(* Logix 5000 AddOnInstructionDefinition export Banner_QS18E_Param_v4; software revision 33.00; part 2 of 3 *)
(* tags used below, declared in another part *)
   QS18E : Banner_QS18E_v4;
   Port_Data : Banner_IOL_Port_v4;
   Port : DINT;
   Sensor_Type : DINT;   // 1 = D, DV, LP, CV, & FP models, 2 = EV or E models, 3 = RV or R models.
   Local_Control : DINT;
   Command_Being_Processed : BOOL;
   Update_Archive : BOOL;
   Index_Write_Inprocess : INT;
   Index_Write_Control : INT;
   Inprocess_Index : DINT;
(* Banner_QS18E_Param_v4, continued *)

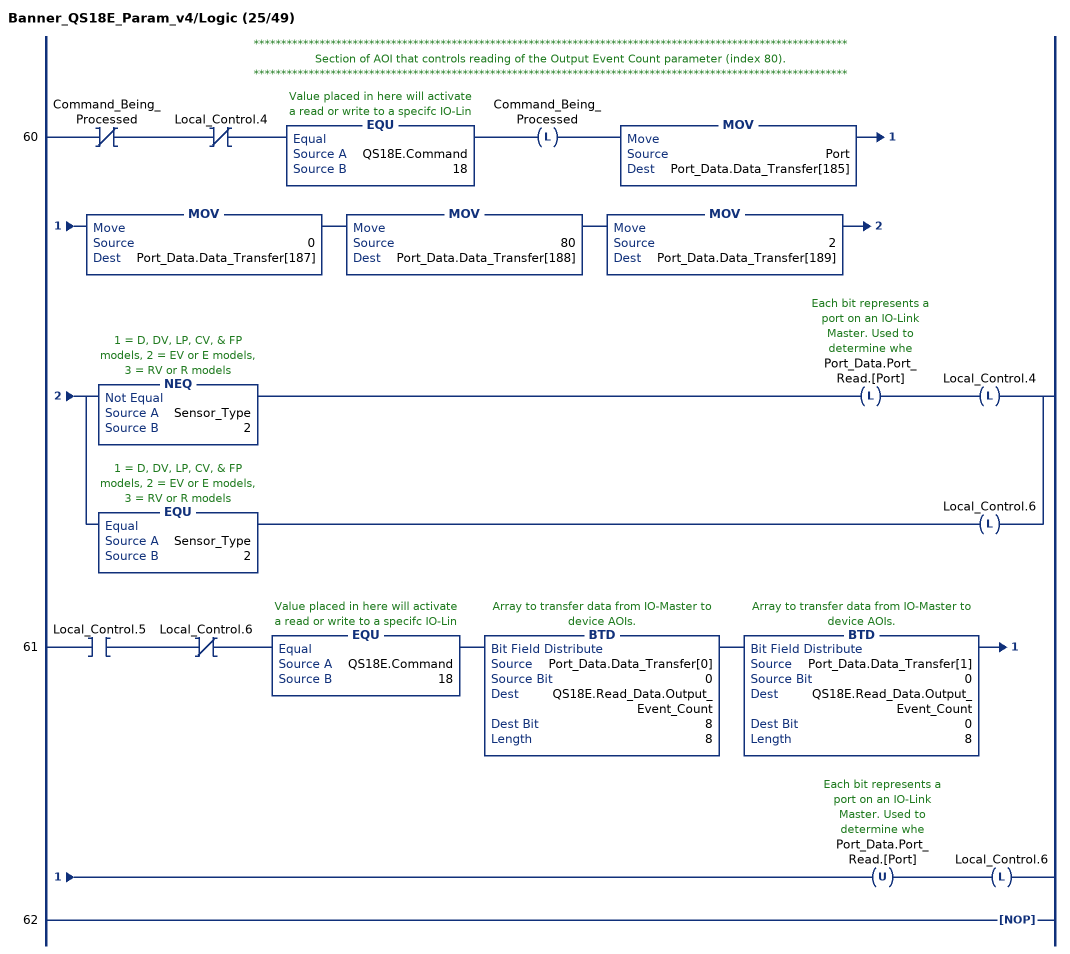
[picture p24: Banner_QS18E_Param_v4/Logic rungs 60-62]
   // ************************************************************************************************************
   // Section of AOI that controls reading of the Output Event Count parameter (index 80).
   // ************************************************************************************************************
   60: XIO(Command_Being_Processed)XIO(Local_Control.4)EQU(QS18E.Command,18)OTL(Command_Being_Processed)MOV(Port,Port_Data.Data_Transfer[185])MOV(0,Port_Data.Data_Transfer[187])MOV(80,Port_Data.Data_Transfer[188])MOV(2,Port_Data.Data_Transfer[189])[NEQ(Sensor_Type,2) OTL(Port_Data.Port_Read.[Port]) OTL(Local_Control.4) ,EQU(Sensor_Type,2) OTL(Local_Control.6) ];
   61: XIC(Local_Control.5)XIO(Local_Control.6)EQU(QS18E.Command,18)BTD(Port_Data.Data_Transfer[0],0,QS18E.Read_Data.Output_Event_Count,8,8)BTD(Port_Data.Data_Transfer[1],0,QS18E.Read_Data.Output_Event_Count,0,8)OTU(Port_Data.Port_Read.[Port])OTL(Local_Control.6);
   62: NOP();
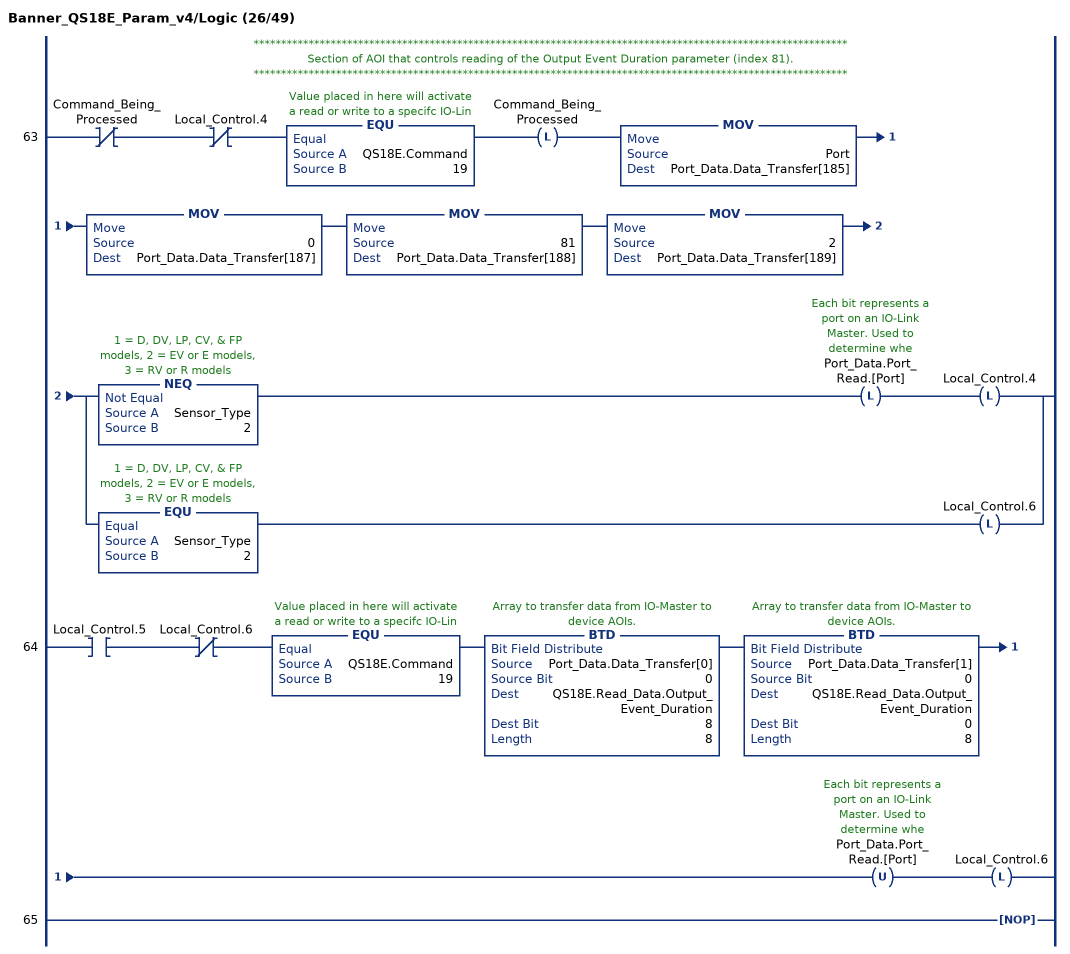
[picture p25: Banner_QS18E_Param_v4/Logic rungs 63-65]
   // ************************************************************************************************************
   // Section of AOI that controls reading of the Output Event Duration parameter (index 81).
   // ************************************************************************************************************
   63: XIO(Command_Being_Processed)XIO(Local_Control.4)EQU(QS18E.Command,19)OTL(Command_Being_Processed)MOV(Port,Port_Data.Data_Transfer[185])MOV(0,Port_Data.Data_Transfer[187])MOV(81,Port_Data.Data_Transfer[188])MOV(2,Port_Data.Data_Transfer[189])[NEQ(Sensor_Type,2) OTL(Port_Data.Port_Read.[Port]) OTL(Local_Control.4) ,EQU(Sensor_Type,2) OTL(Local_Control.6) ];
   64: XIC(Local_Control.5)XIO(Local_Control.6)EQU(QS18E.Command,19)BTD(Port_Data.Data_Transfer[0],0,QS18E.Read_Data.Output_Event_Duration,8,8)BTD(Port_Data.Data_Transfer[1],0,QS18E.Read_Data.Output_Event_Duration,0,8)OTU(Port_Data.Port_Read.[Port])OTL(Local_Control.6);
   65: NOP();
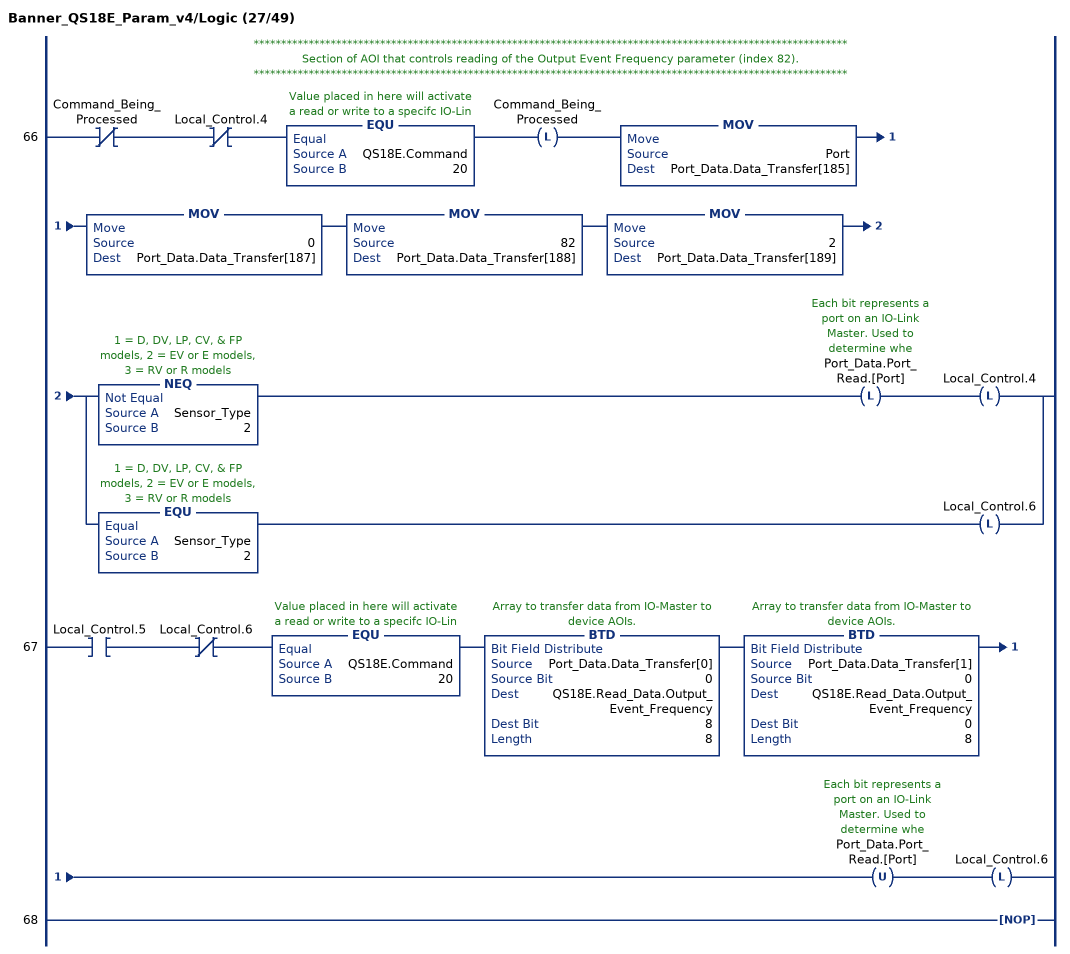
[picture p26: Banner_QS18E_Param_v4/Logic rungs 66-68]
   // ************************************************************************************************************
   // Section of AOI that controls reading of the Output Event Frequency parameter (index 82).
   // ************************************************************************************************************
   66: XIO(Command_Being_Processed)XIO(Local_Control.4)EQU(QS18E.Command,20)OTL(Command_Being_Processed)MOV(Port,Port_Data.Data_Transfer[185])MOV(0,Port_Data.Data_Transfer[187])MOV(82,Port_Data.Data_Transfer[188])MOV(2,Port_Data.Data_Transfer[189])[NEQ(Sensor_Type,2) OTL(Port_Data.Port_Read.[Port]) OTL(Local_Control.4) ,EQU(Sensor_Type,2) OTL(Local_Control.6) ];
   67: XIC(Local_Control.5)XIO(Local_Control.6)EQU(QS18E.Command,20)BTD(Port_Data.Data_Transfer[0],0,QS18E.Read_Data.Output_Event_Frequency,8,8)BTD(Port_Data.Data_Transfer[1],0,QS18E.Read_Data.Output_Event_Frequency,0,8)OTU(Port_Data.Port_Read.[Port])OTL(Local_Control.6);
   68: NOP();
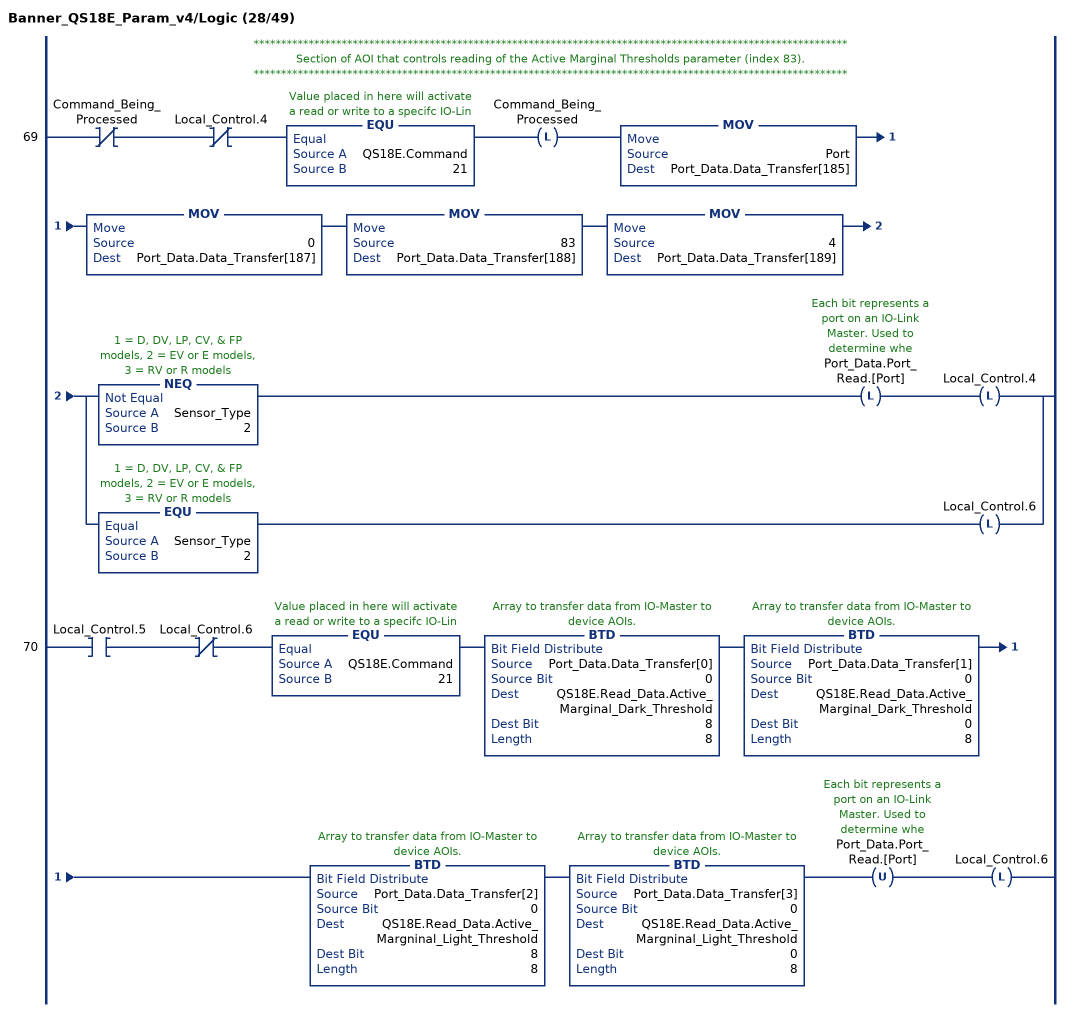
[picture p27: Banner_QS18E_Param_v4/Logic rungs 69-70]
   // ************************************************************************************************************
   // Section of AOI that controls reading of the Active Marginal Thresholds parameter (index 83).
   // ************************************************************************************************************
   69: XIO(Command_Being_Processed)XIO(Local_Control.4)EQU(QS18E.Command,21)OTL(Command_Being_Processed)MOV(Port,Port_Data.Data_Transfer[185])MOV(0,Port_Data.Data_Transfer[187])MOV(83,Port_Data.Data_Transfer[188])MOV(4,Port_Data.Data_Transfer[189])[NEQ(Sensor_Type,2) OTL(Port_Data.Port_Read.[Port]) OTL(Local_Control.4) ,EQU(Sensor_Type,2) OTL(Local_Control.6) ];
   70: XIC(Local_Control.5)XIO(Local_Control.6)EQU(QS18E.Command,21)BTD(Port_Data.Data_Transfer[0],0,QS18E.Read_Data.Active_Marginal_Dark_Threshold,8,8)BTD(Port_Data.Data_Transfer[1],0,QS18E.Read_Data.Active_Marginal_Dark_Threshold,0,8)BTD(Port_Data.Data_Transfer[2],0,QS18E.Read_Data.Active_Margninal_Light_Threshold,8,8)BTD(Port_Data.Data_Transfer[3],0,QS18E.Read_Data.Active_Margninal_Light_Threshold,0,8)OTU(Port_Data.Port_Read.[Port])OTL(Local_Control.6);
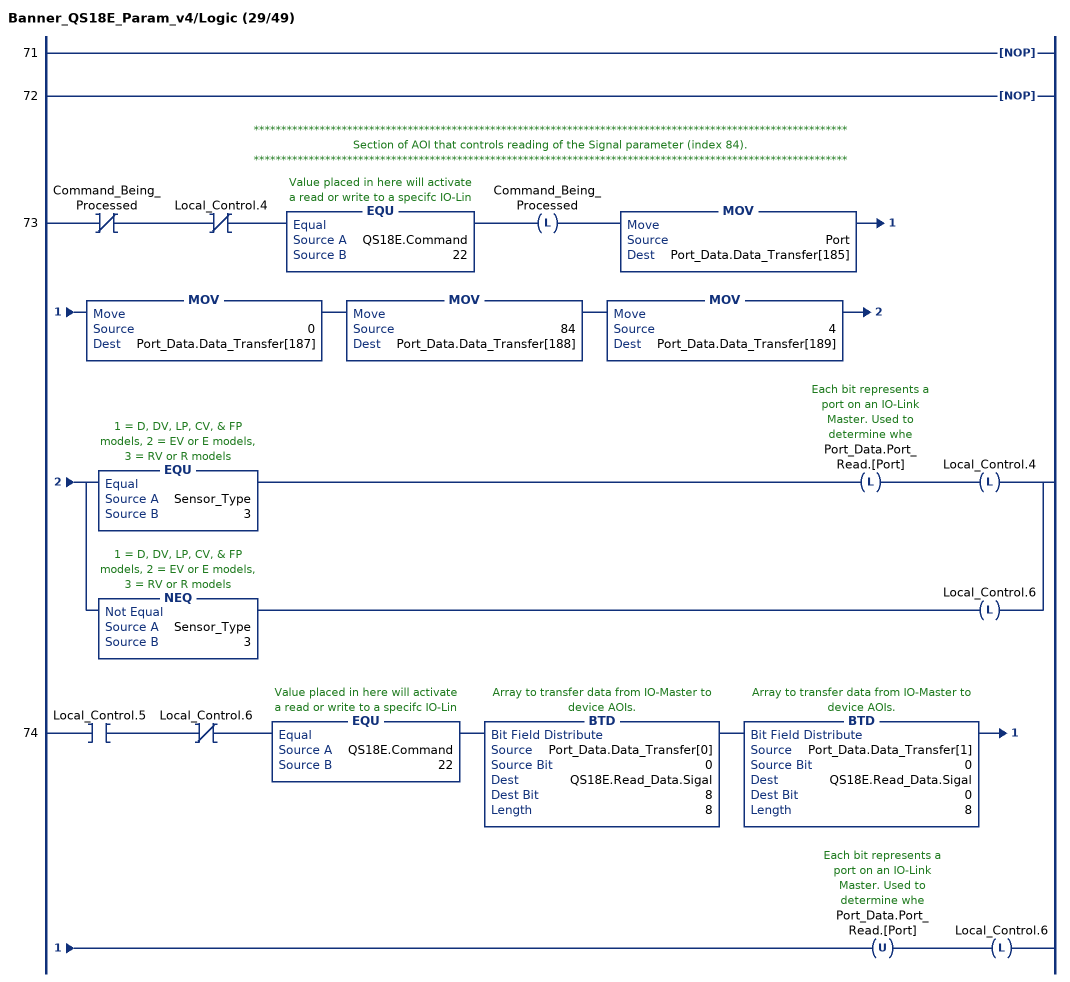
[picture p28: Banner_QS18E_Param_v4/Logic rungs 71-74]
   71: NOP();
   72: NOP();
   // ************************************************************************************************************
   // Section of AOI that controls reading of the Signal parameter (index 84).
   // ************************************************************************************************************
   73: XIO(Command_Being_Processed)XIO(Local_Control.4)EQU(QS18E.Command,22)OTL(Command_Being_Processed)MOV(Port,Port_Data.Data_Transfer[185])MOV(0,Port_Data.Data_Transfer[187])MOV(84,Port_Data.Data_Transfer[188])MOV(4,Port_Data.Data_Transfer[189])[EQU(Sensor_Type,3) OTL(Port_Data.Port_Read.[Port]) OTL(Local_Control.4) ,NEQ(Sensor_Type,3) OTL(Local_Control.6) ];
   74: XIC(Local_Control.5)XIO(Local_Control.6)EQU(QS18E.Command,22)BTD(Port_Data.Data_Transfer[0],0,QS18E.Read_Data.Sigal,8,8)BTD(Port_Data.Data_Transfer[1],0,QS18E.Read_Data.Sigal,0,8)OTU(Port_Data.Port_Read.[Port])OTL(Local_Control.6);
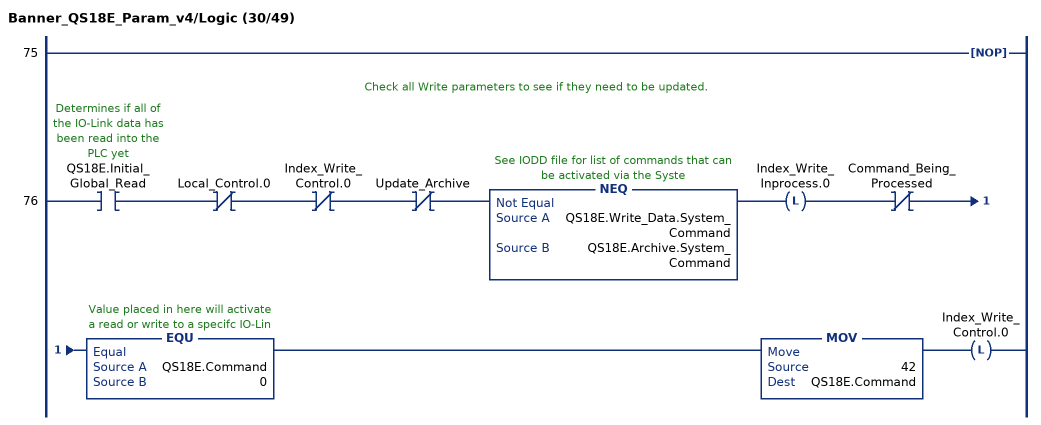
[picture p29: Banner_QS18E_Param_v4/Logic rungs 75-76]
   75: NOP();
   // Check all Write parameters to see if they need to be updated.
   76: XIC(QS18E.Initial_Global_Read)XIO(Local_Control.0)XIO(Index_Write_Control.0)XIO(Update_Archive)NEQ(QS18E.Write_Data.System_Command,QS18E.Archive.System_Command)OTL(Index_Write_Inprocess.0)XIO(Command_Being_Processed)EQU(QS18E.Command,0)MOV(42,QS18E.Command)OTL(Index_Write_Control.0);
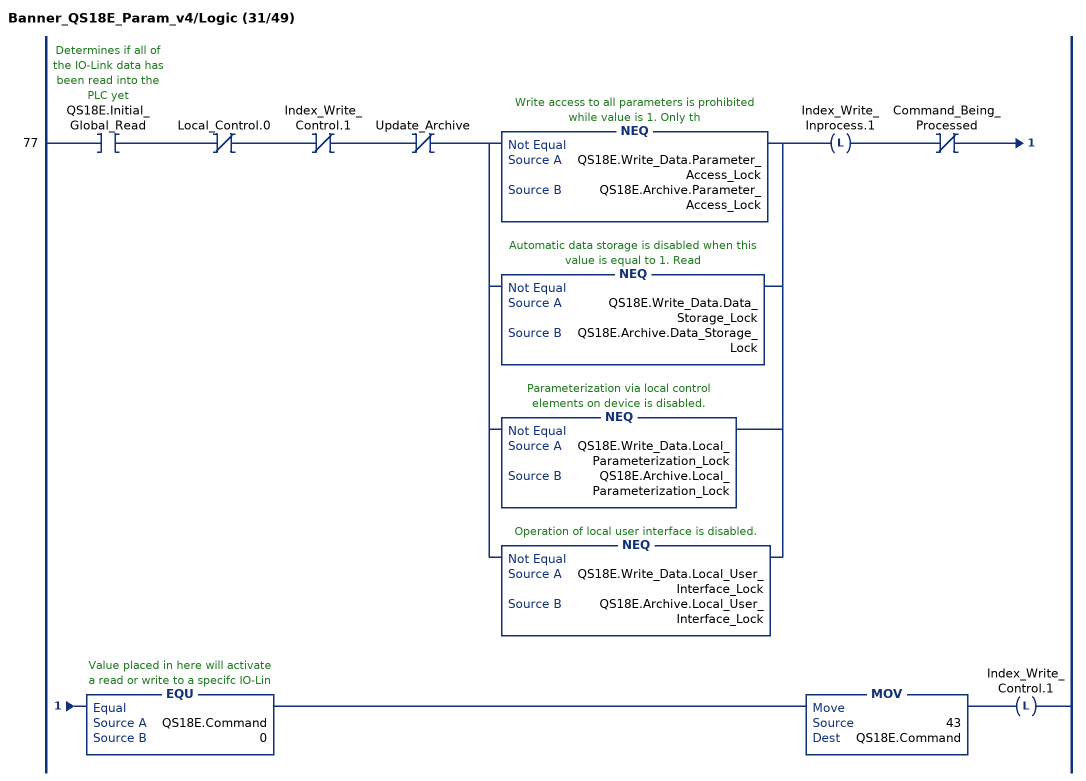
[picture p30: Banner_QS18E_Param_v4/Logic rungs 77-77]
   77: XIC(QS18E.Initial_Global_Read)XIO(Local_Control.0)XIO(Index_Write_Control.1)XIO(Update_Archive)[NEQ(QS18E.Write_Data.Parameter_Access_Lock,QS18E.Archive.Parameter_Access_Lock) ,NEQ(QS18E.Write_Data.Data_Storage_Lock,QS18E.Archive.Data_Storage_Lock) ,NEQ(QS18E.Write_Data.Local_Parameterization_Lock,QS18E.Archive.Local_Parameterization_Lock) ,NEQ(QS18E.Write_Data.Local_User_Interface_Lock,QS18E.Archive.Local_User_Interface_Lock) ]OTL(Index_Write_Inprocess.1)XIO(Command_Being_Processed)EQU(QS18E.Command,0)MOV(43,QS18E.Command)OTL(Index_Write_Control.1);
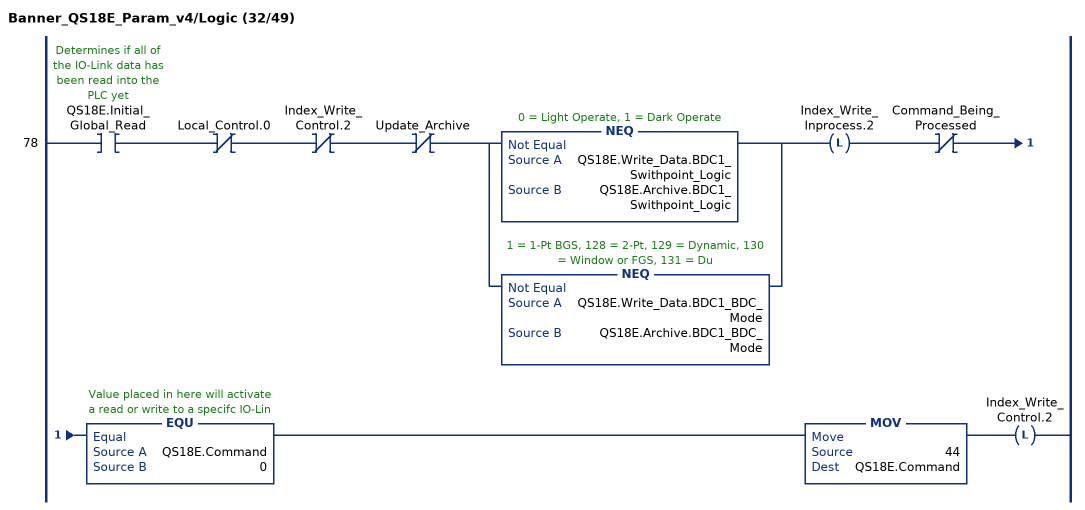
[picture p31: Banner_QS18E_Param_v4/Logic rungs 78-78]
   78: XIC(QS18E.Initial_Global_Read)XIO(Local_Control.0)XIO(Index_Write_Control.2)XIO(Update_Archive)[NEQ(QS18E.Write_Data.BDC1_Swithpoint_Logic,QS18E.Archive.BDC1_Swithpoint_Logic) ,NEQ(QS18E.Write_Data.BDC1_BDC_Mode,QS18E.Archive.BDC1_BDC_Mode) ]OTL(Index_Write_Inprocess.2)XIO(Command_Being_Processed)EQU(QS18E.Command,0)MOV(44,QS18E.Command)OTL(Index_Write_Control.2);
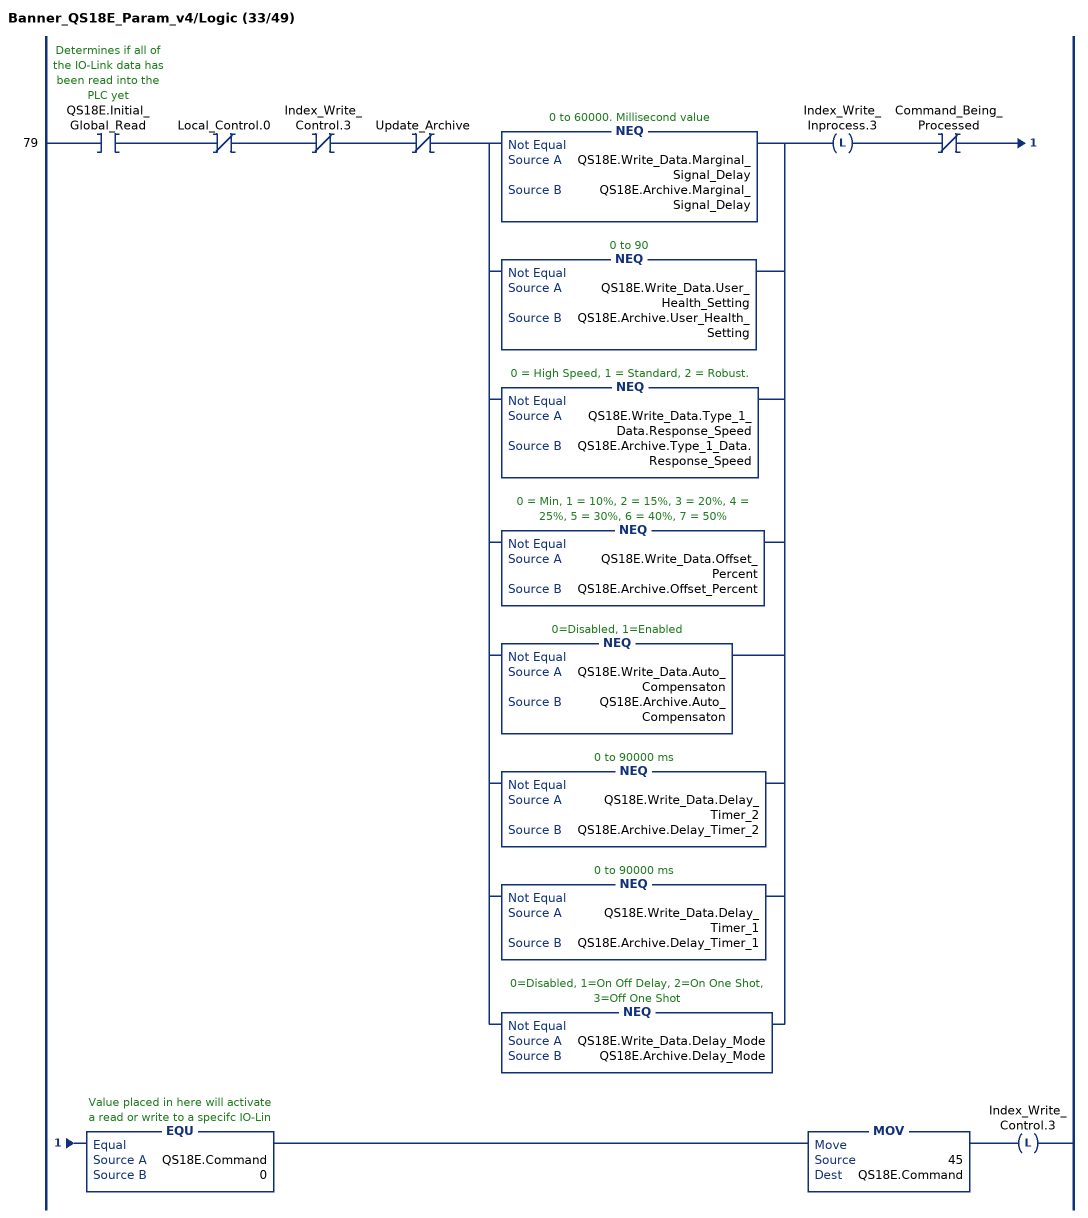
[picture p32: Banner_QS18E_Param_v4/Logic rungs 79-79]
   79: XIC(QS18E.Initial_Global_Read)XIO(Local_Control.0)XIO(Index_Write_Control.3)XIO(Update_Archive)[NEQ(QS18E.Write_Data.Marginal_Signal_Delay,QS18E.Archive.Marginal_Signal_Delay) ,NEQ(QS18E.Write_Data.User_Health_Setting,QS18E.Archive.User_Health_Setting) ,NEQ(QS18E.Write_Data.Type_1_Data.Response_Speed,QS18E.Archive.Type_1_Data.Response_Speed) ,NEQ(QS18E.Write_Data.Offset_Percent,QS18E.Archive.Offset_Percent) ,NEQ(QS18E.Write_Data.Auto_Compensaton,QS18E.Archive.Auto_Compensaton) ,NEQ(QS18E.Write_Data.Delay_Timer_2,QS18E.Archive.Delay_Timer_2) ,NEQ(QS18E.Write_Data.Delay_Timer_1,QS18E.Archive.Delay_Timer_1) ,NEQ(QS18E.Write_Data.Delay_Mode,QS18E.Archive.Delay_Mode) ]OTL(Index_Write_Inprocess.3)XIO(Command_Being_Processed)EQU(QS18E.Command,0)MOV(45,QS18E.Command)OTL(Index_Write_Control.3);
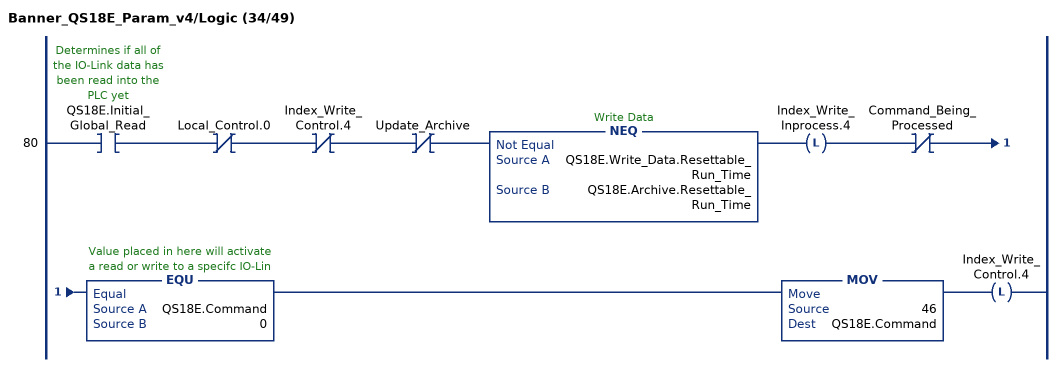
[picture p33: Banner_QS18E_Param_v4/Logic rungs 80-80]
   80: XIC(QS18E.Initial_Global_Read)XIO(Local_Control.0)XIO(Index_Write_Control.4)XIO(Update_Archive)NEQ(QS18E.Write_Data.Resettable_Run_Time,QS18E.Archive.Resettable_Run_Time)OTL(Index_Write_Inprocess.4)XIO(Command_Being_Processed)EQU(QS18E.Command,0)MOV(46,QS18E.Command)OTL(Index_Write_Control.4);
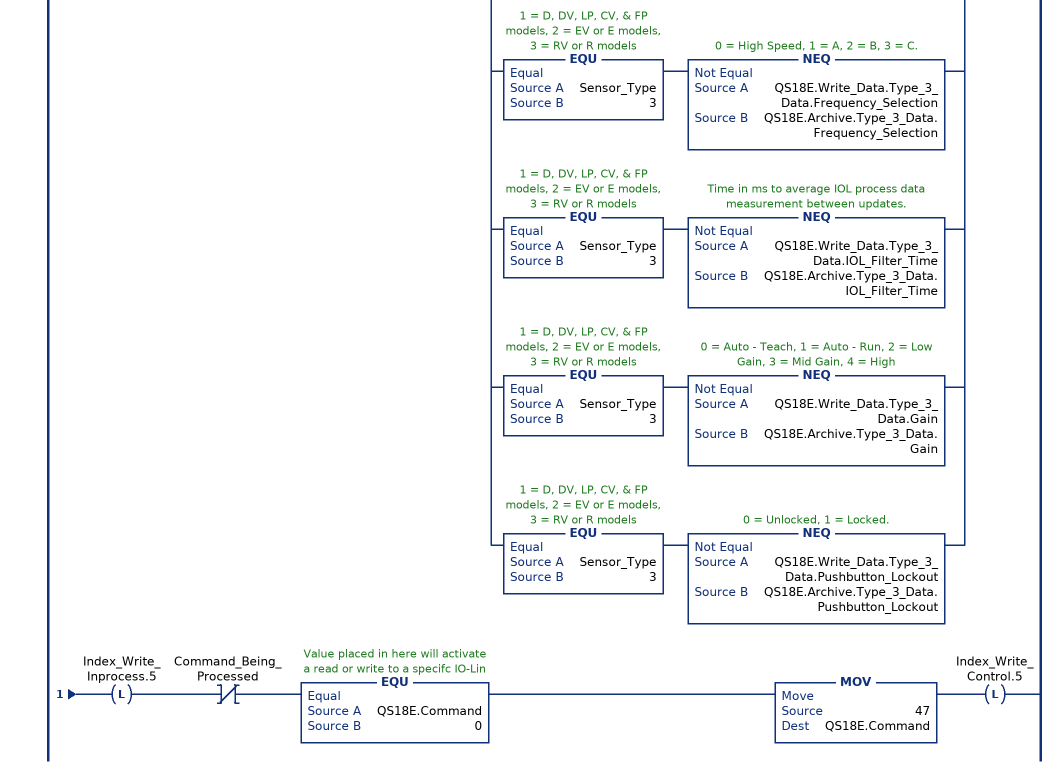
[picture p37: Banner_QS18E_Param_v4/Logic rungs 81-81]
   81: XIC(QS18E.Initial_Global_Read)XIO(Local_Control.0)XIO(Index_Write_Control.5)XIO(Update_Archive)[EQU(Sensor_Type,1) NEQ(QS18E.Write_Data.Type_1_Data.Polarity_of_Pins_2_and_4,QS18E.Archive.Type_1_Data.Polarity_of_Pins_2_and_4) ,EQU(Sensor_Type,1) NEQ(QS18E.Write_Data.Type_1_Data.Pin_2_Config,QS18E.Archive.Type_1_Data.Pin_2_Config) ,EQU(Sensor_Type,1) NEQ(QS18E.Write_Data.Type_1_Data.Process_Data_Input_Config,QS18E.Archive.Type_1_Data.Process_Data_Input_Config) ,EQU(Sensor_Type,1) NEQ(QS18E.Write_Data.Type_1_Data.Marginal_Mode,QS18E.Archive.Type_1_Data.Marginal_Mode) ,EQU(Sensor_Type,1) NEQ(QS18E.Write_Data.Type_1_Data.User_Marginal_Light,QS18E.Archive.Type_1_Data.User_Marginal_Light) ,EQU(Sensor_Type,1) NEQ(QS18E.Write_Data.Type_1_Data.User_Marginal_Dark,QS18E.Archive.Type_1_Data.User_Marginal_Dark) ,EQU(Sensor_Type,1) NEQ(QS18E.Write_Data.Type_1_Data.LED_Power,QS18E.Archive.Type_1_Data.LED_Power) ,EQU(Sensor_Type,2) NEQ(QS18E.Write_Data.Type_2_Data.Polarity_of_Pins_2_and_4,QS18E.Archive.Type_2_Data.Polarity_of_Pins_2_and_4) ,EQU(Sensor_Type,2) NEQ(QS18E.Write_Data.Type_2_Data.Pin_2_Config,QS18E.Archive.Type_2_Data.Pin_2_Config) ,EQU(Sensor_Type,2) NEQ(QS18E.Write_Data.Type_2_Data.Frequency_Selection,QS18E.Archive.Type_2_Data.Frequency_Selection) ,EQU(Sensor_Type,2) NEQ(QS18E.Write_Data.Type_2_Data.Power_Level,QS18E.Archive.Type_2_Data.Power_Level) ,EQU(Sensor_Type,2) NEQ(QS18E.Write_Data.Type_2_Data.Pushbutton_Lockout,QS18E.Archive.Type_2_Data.Pushbutton_Lockout) ,EQU(Sensor_Type,3) NEQ(QS18E.Write_Data.Type_3_Data.Polarity_of_Pins_2_and_4,QS18E.Archive.Type_3_Data.Polarity_of_Pins_2_and_4) ,EQU(Sensor_Type,3) NEQ(QS18E.Write_Data.Type_3_Data.Pin_2_Config,QS18E.Archive.Type_3_Data.Pin_2_Config) ,EQU(Sensor_Type,3) NEQ(QS18E.Write_Data.Type_3_Data.Process_Data_Input_Config,QS18E.Archive.Type_3_Data.Process_Data_Input_Config) ,EQU(Sensor_Type,3) NEQ(QS18E.Write_Data.Type_3_Data.Marginal_Mode,QS18E.Archive.Type_3_Data.Marginal_Mode) ,EQU(Sensor_Type,3) NEQ(QS18E.Write_Data.Type_3_Data.User_Marginal_Light,QS18E.Archive.Type_3_Data.User_Marginal_Light) ,EQU(Sensor_Type,3) NEQ(QS18E.Write_Data.Type_3_Data.User_Marginal_Dark,QS18E.Archive.Type_3_Data.User_Marginal_Dark) ,EQU(Sensor_Type,3) NEQ(QS18E.Write_Data.Type_3_Data.Frequency_Selection,QS18E.Archive.Type_3_Data.Frequency_Selection) ,EQU(Sensor_Type,3) NEQ(QS18E.Write_Data.Type_3_Data.IOL_Filter_Time,QS18E.Archive.Type_3_Data.IOL_Filter_Time) ,EQU(Sensor_Type,3) NEQ(QS18E.Write_Data.Type_3_Data.Gain,QS18E.Archive.Type_3_Data.Gain) ,EQU(Sensor_Type,3) NEQ(QS18E.Write_Data.Type_3_Data.Pushbutton_Lockout,QS18E.Archive.Type_3_Data.Pushbutton_Lockout) ]OTL(Index_Write_Inprocess.5)XIO(Command_Being_Processed)EQU(QS18E.Command,0)MOV(47,QS18E.Command)OTL(Index_Write_Control.5);
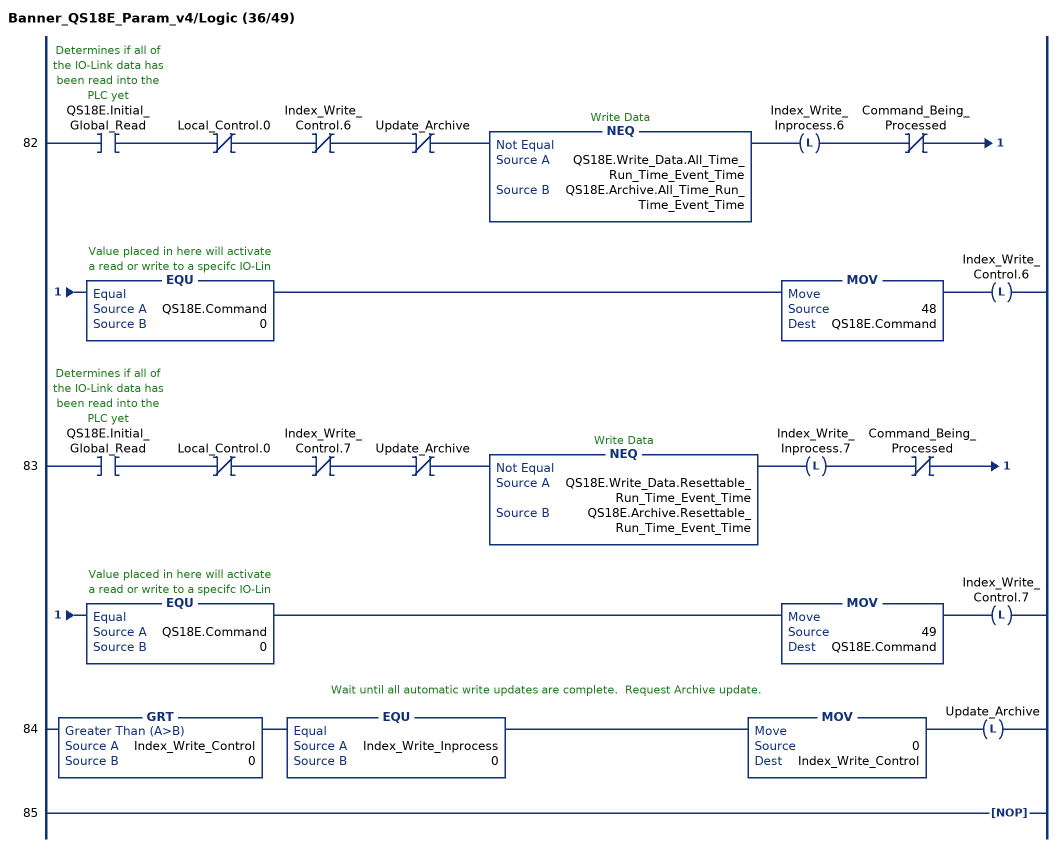
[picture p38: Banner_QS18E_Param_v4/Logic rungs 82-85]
   82: XIC(QS18E.Initial_Global_Read)XIO(Local_Control.0)XIO(Index_Write_Control.6)XIO(Update_Archive)NEQ(QS18E.Write_Data.All_Time_Run_Time_Event_Time,QS18E.Archive.All_Time_Run_Time_Event_Time)OTL(Index_Write_Inprocess.6)XIO(Command_Being_Processed)EQU(QS18E.Command,0)MOV(48,QS18E.Command)OTL(Index_Write_Control.6);
   83: XIC(QS18E.Initial_Global_Read)XIO(Local_Control.0)XIO(Index_Write_Control.7)XIO(Update_Archive)NEQ(QS18E.Write_Data.Resettable_Run_Time_Event_Time,QS18E.Archive.Resettable_Run_Time_Event_Time)OTL(Index_Write_Inprocess.7)XIO(Command_Being_Processed)EQU(QS18E.Command,0)MOV(49,QS18E.Command)OTL(Index_Write_Control.7);
   // Wait until all automatic write updates are complete.  Request Archive update.
   84: GRT(Index_Write_Control,0)EQU(Index_Write_Inprocess,0)MOV(0,Index_Write_Control)OTL(Update_Archive);
   85: NOP();
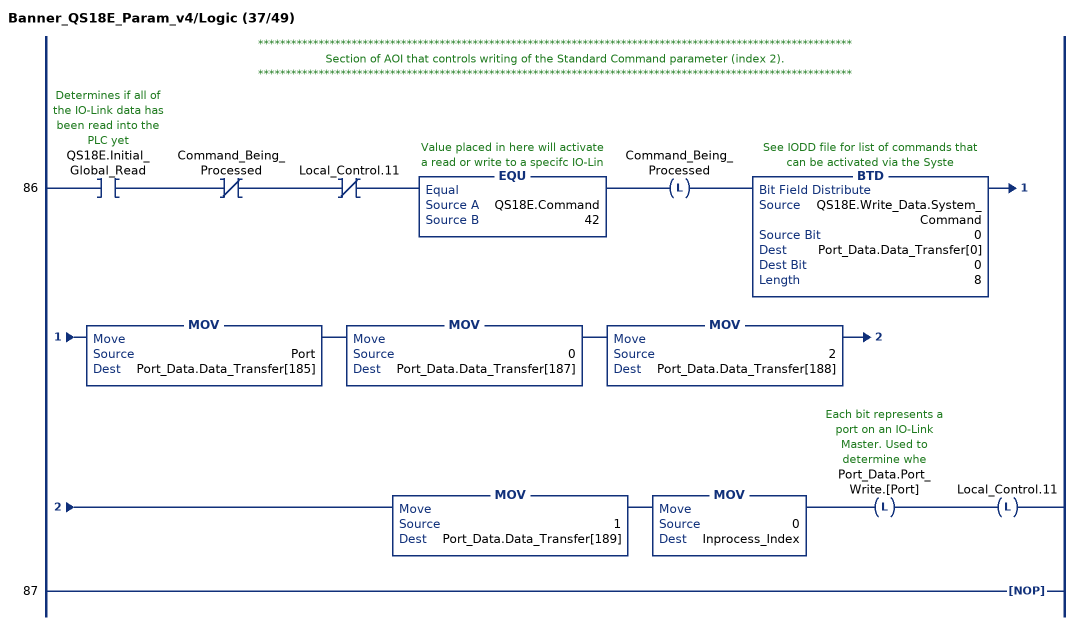
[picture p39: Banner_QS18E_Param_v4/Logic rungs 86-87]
   // ************************************************************************************************************
   // Section of AOI that controls writing of the Standard Command parameter (index 2).
   // ************************************************************************************************************
   86: XIC(QS18E.Initial_Global_Read)XIO(Command_Being_Processed)XIO(Local_Control.11)EQU(QS18E.Command,42)OTL(Command_Being_Processed)BTD(QS18E.Write_Data.System_Command,0,Port_Data.Data_Transfer[0],0,8)MOV(Port,Port_Data.Data_Transfer[185])MOV(0,Port_Data.Data_Transfer[187])MOV(2,Port_Data.Data_Transfer[188])MOV(1,Port_Data.Data_Transfer[189])MOV(0,Inprocess_Index)OTL(Port_Data.Port_Write.[Port])OTL(Local_Control.11);
   87: NOP();
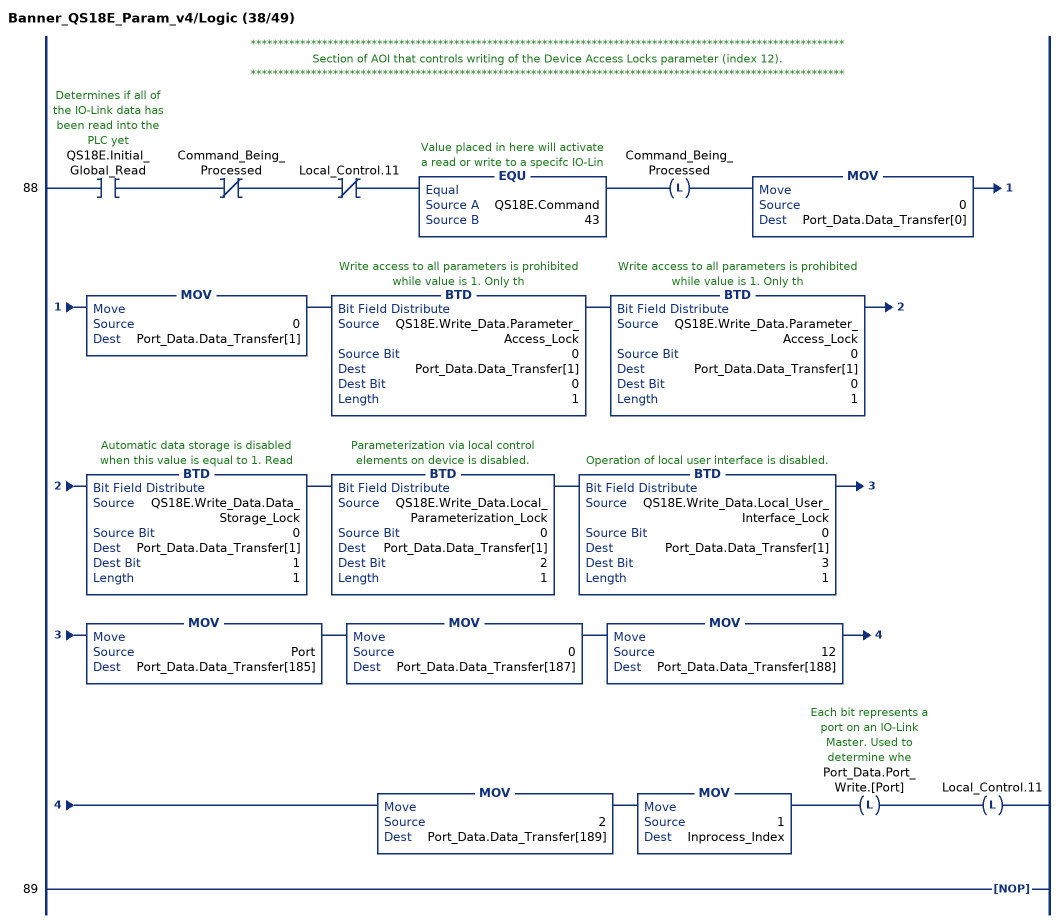
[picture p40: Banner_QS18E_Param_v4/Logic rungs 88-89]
   // ************************************************************************************************************
   // Section of AOI that controls writing of the Device Access Locks parameter (index 12).
   // ************************************************************************************************************
   88: XIC(QS18E.Initial_Global_Read)XIO(Command_Being_Processed)XIO(Local_Control.11)EQU(QS18E.Command,43)OTL(Command_Being_Processed)MOV(0,Port_Data.Data_Transfer[0])MOV(0,Port_Data.Data_Transfer[1])BTD(QS18E.Write_Data.Parameter_Access_Lock,0,Port_Data.Data_Transfer[1],0,1)BTD(QS18E.Write_Data.Parameter_Access_Lock,0,Port_Data.Data_Transfer[1],0,1)BTD(QS18E.Write_Data.Data_Storage_Lock,0,Port_Data.Data_Transfer[1],1,1)BTD(QS18E.Write_Data.Local_Parameterization_Lock,0,Port_Data.Data_Transfer[1],2,1)BTD(QS18E.Write_Data.Local_User_Interface_Lock,0,Port_Data.Data_Transfer[1],3,1)MOV(Port,Port_Data.Data_Transfer[185])MOV(0,Port_Data.Data_Transfer[187])MOV(12,Port_Data.Data_Transfer[188])MOV(2,Port_Data.Data_Transfer[189])MOV(1,Inprocess_Index)OTL(Port_Data.Port_Write.[Port])OTL(Local_Control.11);
   89: NOP();
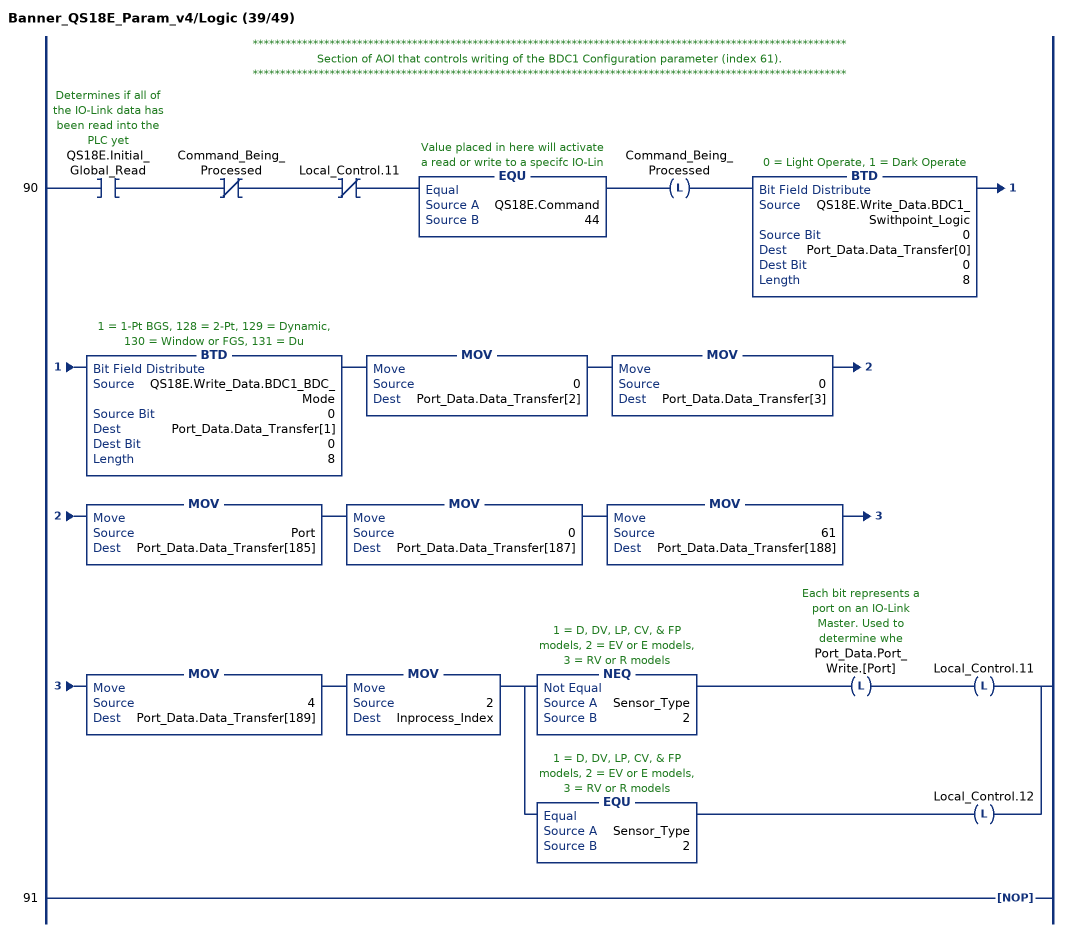
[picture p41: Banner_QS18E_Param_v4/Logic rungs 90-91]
   // ************************************************************************************************************
   // Section of AOI that controls writing of the BDC1 Configuration parameter (index 61).
   // ************************************************************************************************************
   90: XIC(QS18E.Initial_Global_Read)XIO(Command_Being_Processed)XIO(Local_Control.11)EQU(QS18E.Command,44)OTL(Command_Being_Processed)BTD(QS18E.Write_Data.BDC1_Swithpoint_Logic,0,Port_Data.Data_Transfer[0],0,8)BTD(QS18E.Write_Data.BDC1_BDC_Mode,0,Port_Data.Data_Transfer[1],0,8)MOV(0,Port_Data.Data_Transfer[2])MOV(0,Port_Data.Data_Transfer[3])MOV(Port,Port_Data.Data_Transfer[185])MOV(0,Port_Data.Data_Transfer[187])MOV(61,Port_Data.Data_Transfer[188])MOV(4,Port_Data.Data_Transfer[189])MOV(2,Inprocess_Index)[NEQ(Sensor_Type,2) OTL(Port_Data.Port_Write.[Port]) OTL(Local_Control.11) ,EQU(Sensor_Type,2) OTL(Local_Control.12) ];
   91: NOP();
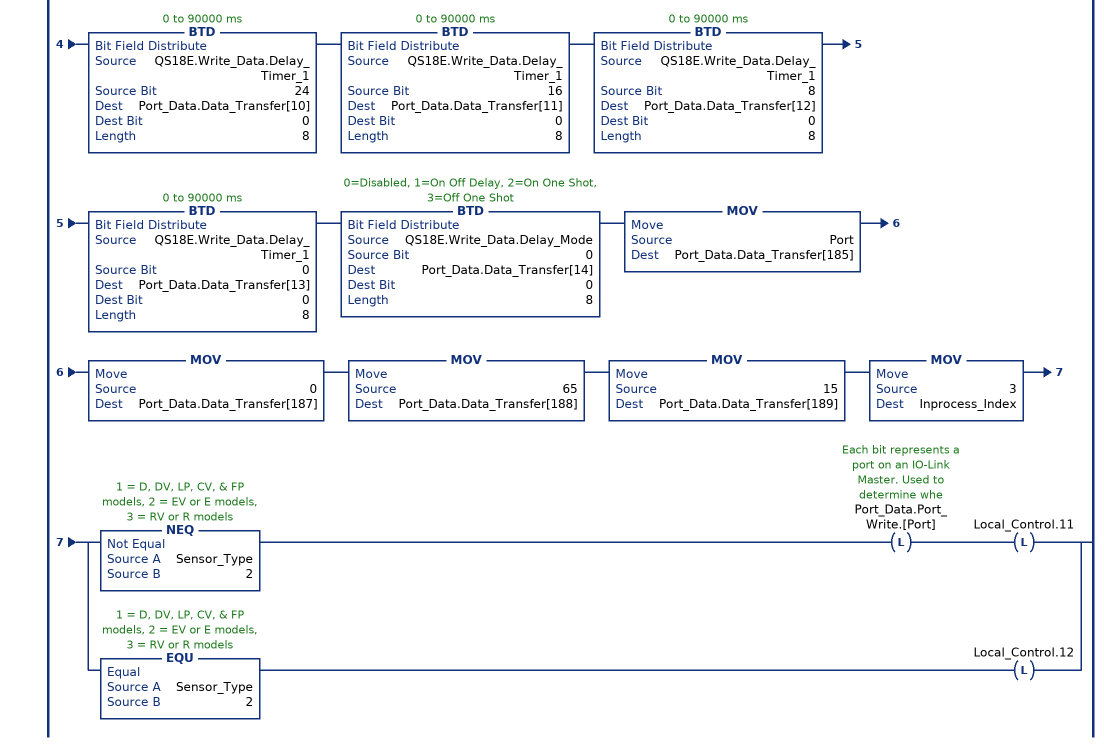
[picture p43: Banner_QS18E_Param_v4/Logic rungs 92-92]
   // ************************************************************************************************************
   // Section of AOI that controls writing of the BDC1 Vendor Specific Configuration parameter (index 65).
   // ************************************************************************************************************
   92: XIC(QS18E.Initial_Global_Read)XIO(Command_Being_Processed)XIO(Local_Control.11)EQU(QS18E.Command,45)OTL(Command_Being_Processed)BTD(QS18E.Write_Data.Marginal_Signal_Delay,8,Port_Data.Data_Transfer[0],0,8)BTD(QS18E.Write_Data.Marginal_Signal_Delay,0,Port_Data.Data_Transfer[1],0,8)BTD(QS18E.Write_Data.User_Health_Setting,0,Port_Data.Data_Transfer[2],0,8)[EQU(Sensor_Type,1) BTD(QS18E.Write_Data.Type_1_Data.Response_Speed,0,Port_Data.Data_Transfer[3],0,8) ,NEQ(Sensor_Type,1) MOV(0,Port_Data.Data_Transfer[3]) ]BTD(QS18E.Write_Data.Offset_Percent,0,Port_Data.Data_Transfer[4],0,8)BTD(QS18E.Write_Data.Auto_Compensaton,0,Port_Data.Data_Transfer[5],0,8)BTD(QS18E.Write_Data.Delay_Timer_2,24,Port_Data.Data_Transfer[6],0,8)BTD(QS18E.Write_Data.Delay_Timer_2,16,Port_Data.Data_Transfer[7],0,8)BTD(QS18E.Write_Data.Delay_Timer_2,8,Port_Data.Data_Transfer[8],0,8)BTD(QS18E.Write_Data.Delay_Timer_2,0,Port_Data.Data_Transfer[9],0,8)BTD(QS18E.Write_Data.Delay_Timer_1,24,Port_Data.Data_Transfer[10],0,8)BTD(QS18E.Write_Data.Delay_Timer_1,16,Port_Data.Data_Transfer[11],0,8)BTD(QS18E.Write_Data.Delay_Timer_1,8,Port_Data.Data_Transfer[12],0,8)BTD(QS18E.Write_Data.Delay_Timer_1,0,Port_Data.Data_Transfer[13],0,8)BTD(QS18E.Write_Data.Delay_Mode,0,Port_Data.Data_Transfer[14],0,8)MOV(Port,Port_Data.Data_Transfer[185])MOV(0,Port_Data.Data_Transfer[187])MOV(65,Port_Data.Data_Transfer[188])MOV(15,Port_Data.Data_Transfer[189])MOV(3,Inprocess_Index)[NEQ(Sensor_Type,2) OTL(Port_Data.Port_Write.[Port]) OTL(Local_Control.11) ,EQU(Sensor_Type,2) OTL(Local_Control.12) ];
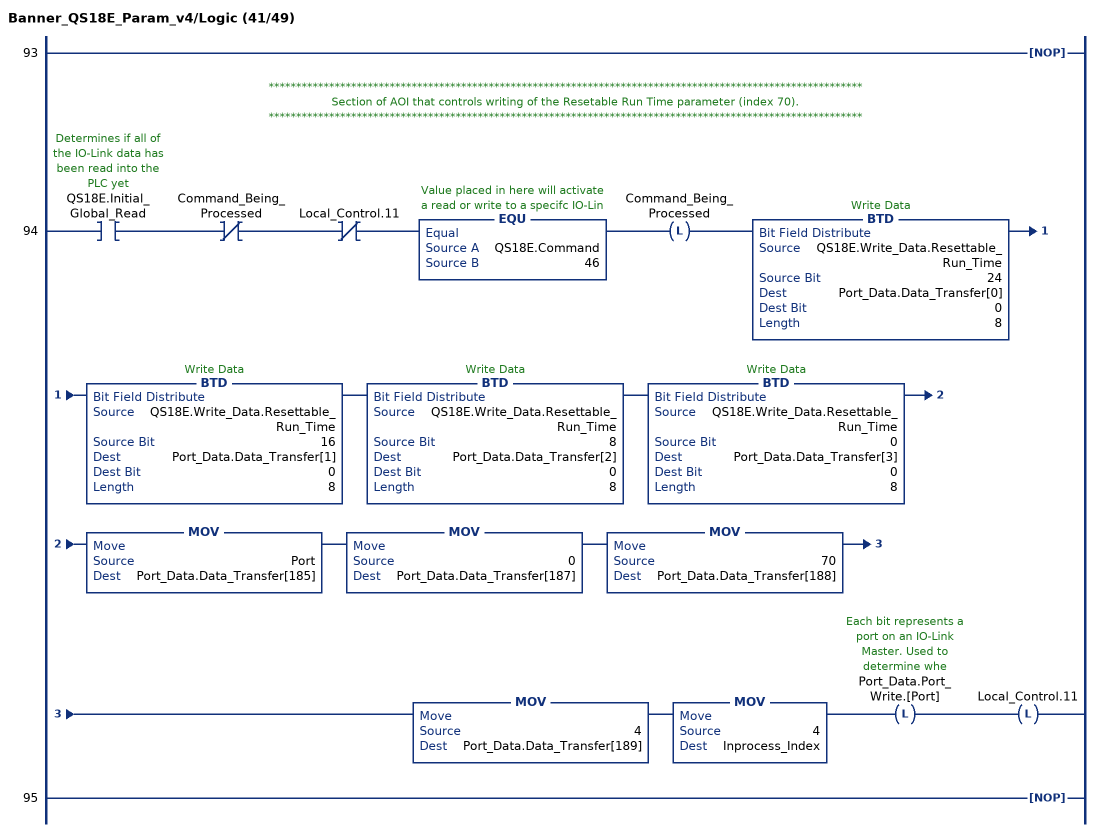
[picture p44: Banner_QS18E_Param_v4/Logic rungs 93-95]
   93: NOP();
   // ************************************************************************************************************
   // Section of AOI that controls writing of the Resetable Run Time parameter (index 70).
   // ************************************************************************************************************
   94: XIC(QS18E.Initial_Global_Read)XIO(Command_Being_Processed)XIO(Local_Control.11)EQU(QS18E.Command,46)OTL(Command_Being_Processed)BTD(QS18E.Write_Data.Resettable_Run_Time,24,Port_Data.Data_Transfer[0],0,8)BTD(QS18E.Write_Data.Resettable_Run_Time,16,Port_Data.Data_Transfer[1],0,8)BTD(QS18E.Write_Data.Resettable_Run_Time,8,Port_Data.Data_Transfer[2],0,8)BTD(QS18E.Write_Data.Resettable_Run_Time,0,Port_Data.Data_Transfer[3],0,8)MOV(Port,Port_Data.Data_Transfer[185])MOV(0,Port_Data.Data_Transfer[187])MOV(70,Port_Data.Data_Transfer[188])MOV(4,Port_Data.Data_Transfer[189])MOV(4,Inprocess_Index)OTL(Port_Data.Port_Write.[Port])OTL(Local_Control.11);
   95: NOP();
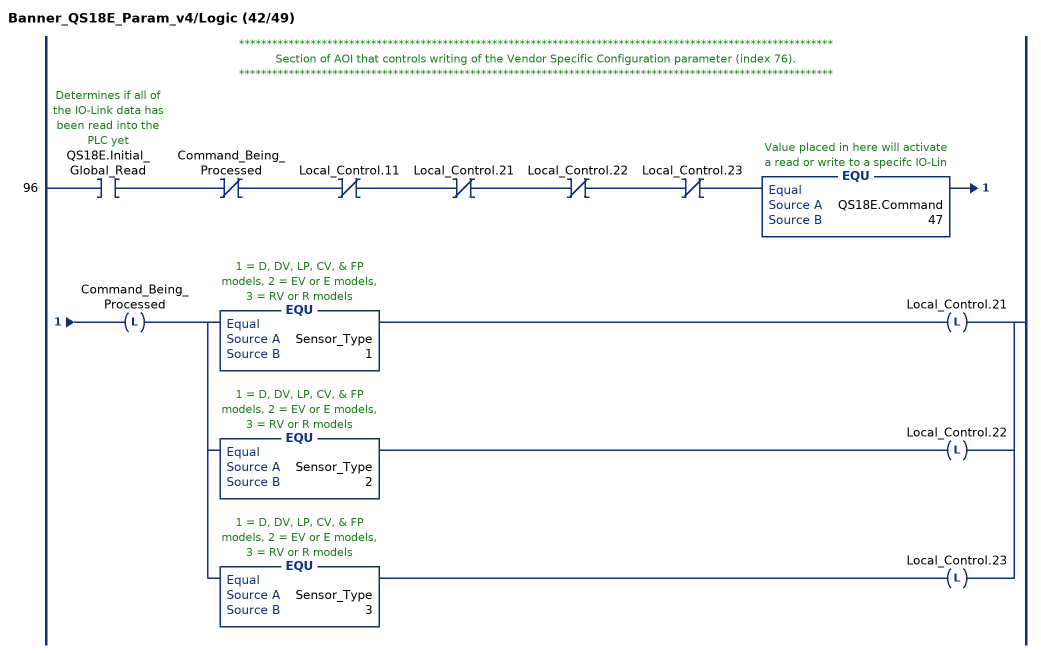
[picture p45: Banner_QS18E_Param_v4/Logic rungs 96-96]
   // ************************************************************************************************************
   // Section of AOI that controls writing of the Vendor Specific Configuration parameter (index 76).
   // ************************************************************************************************************
   96: XIC(QS18E.Initial_Global_Read)XIO(Command_Being_Processed)XIO(Local_Control.11)XIO(Local_Control.21)XIO(Local_Control.22)XIO(Local_Control.23)EQU(QS18E.Command,47)OTL(Command_Being_Processed)[EQU(Sensor_Type,1) OTL(Local_Control.21) ,EQU(Sensor_Type,2) OTL(Local_Control.22) ,EQU(Sensor_Type,3) OTL(Local_Control.23) ];
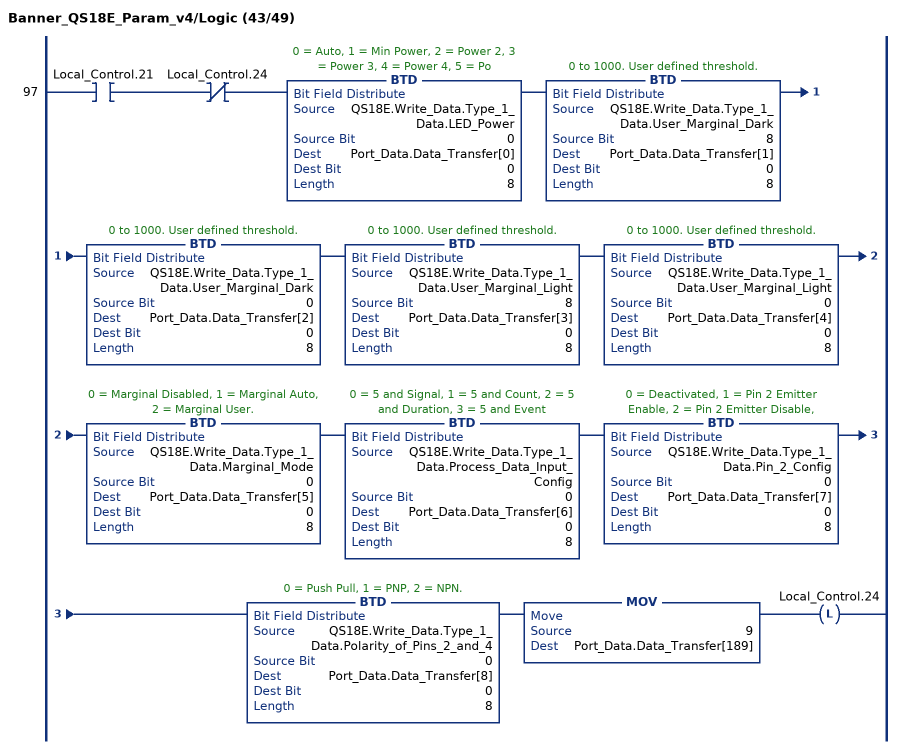
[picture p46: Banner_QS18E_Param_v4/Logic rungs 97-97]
   97: XIC(Local_Control.21)XIO(Local_Control.24)BTD(QS18E.Write_Data.Type_1_Data.LED_Power,0,Port_Data.Data_Transfer[0],0,8)BTD(QS18E.Write_Data.Type_1_Data.User_Marginal_Dark,8,Port_Data.Data_Transfer[1],0,8)BTD(QS18E.Write_Data.Type_1_Data.User_Marginal_Dark,0,Port_Data.Data_Transfer[2],0,8)BTD(QS18E.Write_Data.Type_1_Data.User_Marginal_Light,8,Port_Data.Data_Transfer[3],0,8)BTD(QS18E.Write_Data.Type_1_Data.User_Marginal_Light,0,Port_Data.Data_Transfer[4],0,8)BTD(QS18E.Write_Data.Type_1_Data.Marginal_Mode,0,Port_Data.Data_Transfer[5],0,8)BTD(QS18E.Write_Data.Type_1_Data.Process_Data_Input_Config,0,Port_Data.Data_Transfer[6],0,8)BTD(QS18E.Write_Data.Type_1_Data.Pin_2_Config,0,Port_Data.Data_Transfer[7],0,8)BTD(QS18E.Write_Data.Type_1_Data.Polarity_of_Pins_2_and_4,0,Port_Data.Data_Transfer[8],0,8)MOV(9,Port_Data.Data_Transfer[189])OTL(Local_Control.24);
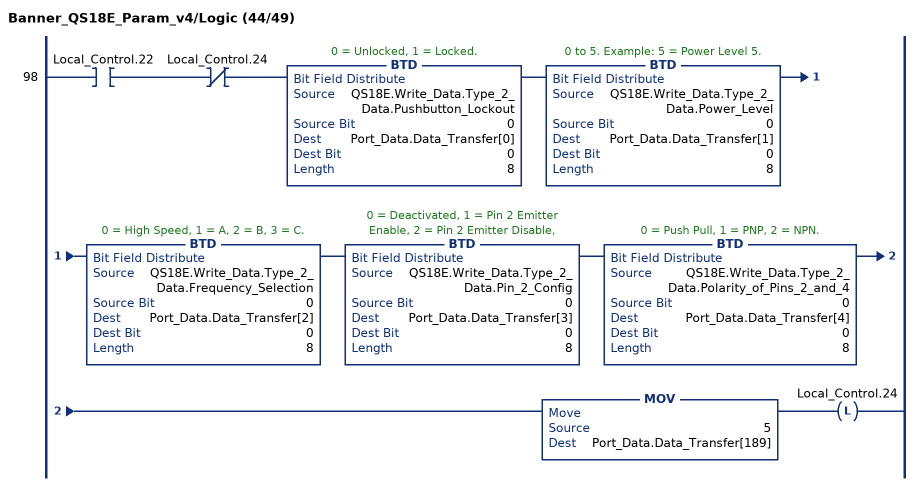
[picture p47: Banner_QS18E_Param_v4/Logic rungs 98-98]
   98: XIC(Local_Control.22)XIO(Local_Control.24)BTD(QS18E.Write_Data.Type_2_Data.Pushbutton_Lockout,0,Port_Data.Data_Transfer[0],0,8)BTD(QS18E.Write_Data.Type_2_Data.Power_Level,0,Port_Data.Data_Transfer[1],0,8)BTD(QS18E.Write_Data.Type_2_Data.Frequency_Selection,0,Port_Data.Data_Transfer[2],0,8)BTD(QS18E.Write_Data.Type_2_Data.Pin_2_Config,0,Port_Data.Data_Transfer[3],0,8)BTD(QS18E.Write_Data.Type_2_Data.Polarity_of_Pins_2_and_4,0,Port_Data.Data_Transfer[4],0,8)MOV(5,Port_Data.Data_Transfer[189])OTL(Local_Control.24);
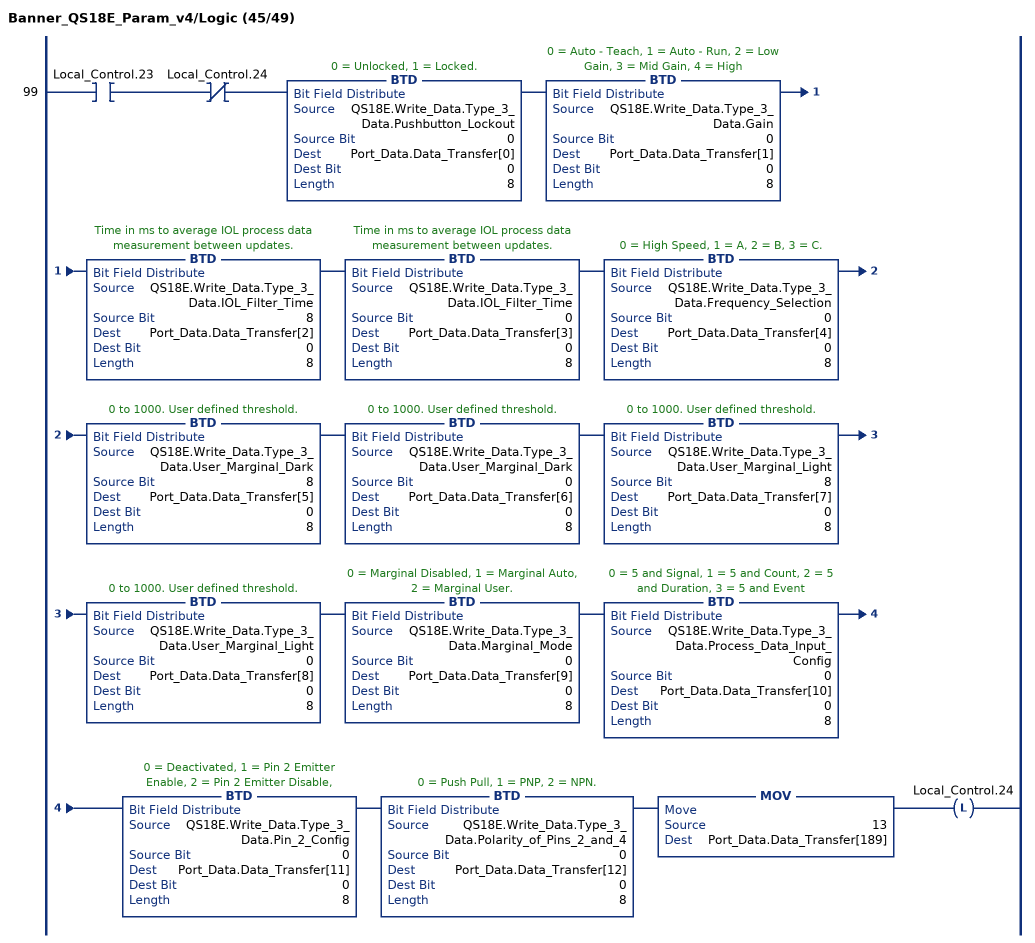
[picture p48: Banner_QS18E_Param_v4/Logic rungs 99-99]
   99: XIC(Local_Control.23)XIO(Local_Control.24)BTD(QS18E.Write_Data.Type_3_Data.Pushbutton_Lockout,0,Port_Data.Data_Transfer[0],0,8)BTD(QS18E.Write_Data.Type_3_Data.Gain,0,Port_Data.Data_Transfer[1],0,8)BTD(QS18E.Write_Data.Type_3_Data.IOL_Filter_Time,8,Port_Data.Data_Transfer[2],0,8)BTD(QS18E.Write_Data.Type_3_Data.IOL_Filter_Time,0,Port_Data.Data_Transfer[3],0,8)BTD(QS18E.Write_Data.Type_3_Data.Frequency_Selection,0,Port_Data.Data_Transfer[4],0,8)BTD(QS18E.Write_Data.Type_3_Data.User_Marginal_Dark,8,Port_Data.Data_Transfer[5],0,8)BTD(QS18E.Write_Data.Type_3_Data.User_Marginal_Dark,0,Port_Data.Data_Transfer[6],0,8)BTD(QS18E.Write_Data.Type_3_Data.User_Marginal_Light,8,Port_Data.Data_Transfer[7],0,8)BTD(QS18E.Write_Data.Type_3_Data.User_Marginal_Light,0,Port_Data.Data_Transfer[8],0,8)BTD(QS18E.Write_Data.Type_3_Data.Marginal_Mode,0,Port_Data.Data_Transfer[9],0,8)BTD(QS18E.Write_Data.Type_3_Data.Process_Data_Input_Config,0,Port_Data.Data_Transfer[10],0,8)BTD(QS18E.Write_Data.Type_3_Data.Pin_2_Config,0,Port_Data.Data_Transfer[11],0,8)BTD(QS18E.Write_Data.Type_3_Data.Polarity_of_Pins_2_and_4,0,Port_Data.Data_Transfer[12],0,8)MOV(13,Port_Data.Data_Transfer[189])OTL(Local_Control.24);
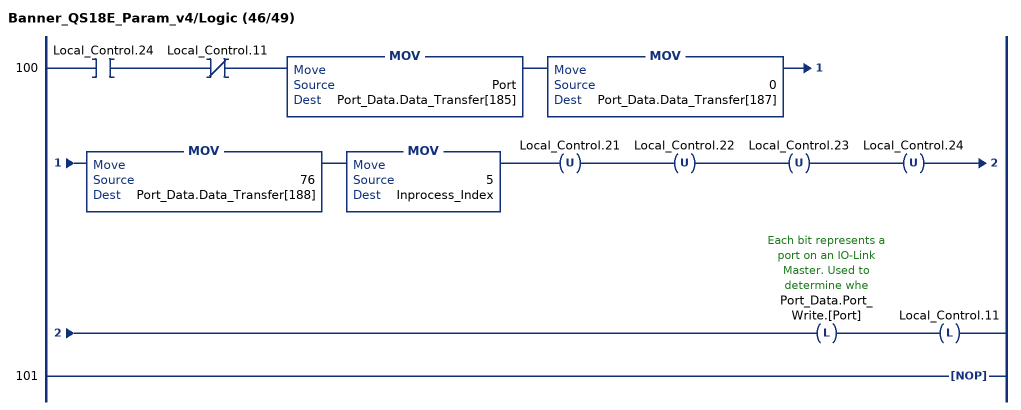
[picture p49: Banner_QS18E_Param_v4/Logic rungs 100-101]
   100: XIC(Local_Control.24)XIO(Local_Control.11)MOV(Port,Port_Data.Data_Transfer[185])MOV(0,Port_Data.Data_Transfer[187])MOV(76,Port_Data.Data_Transfer[188])MOV(5,Inprocess_Index)OTU(Local_Control.21)OTU(Local_Control.22)OTU(Local_Control.23)OTU(Local_Control.24)OTL(Port_Data.Port_Write.[Port])OTL(Local_Control.11);
   101: NOP();
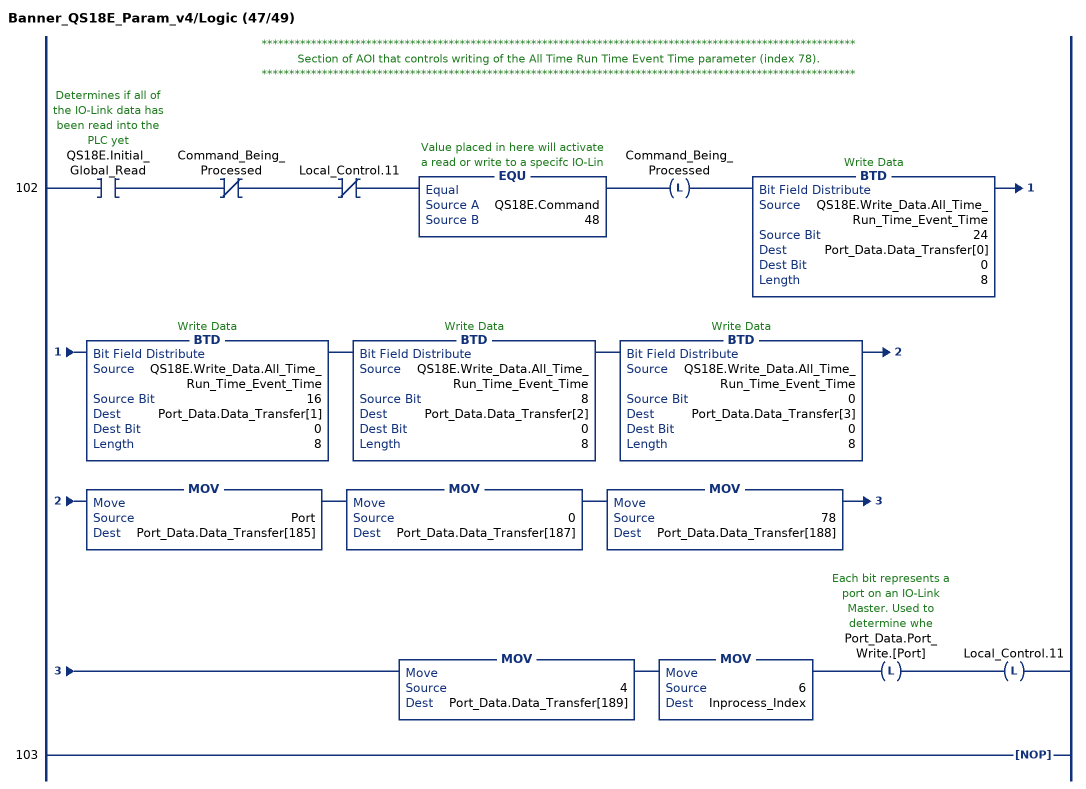
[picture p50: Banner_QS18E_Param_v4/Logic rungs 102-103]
   // ************************************************************************************************************
   // Section of AOI that controls writing of the All Time Run Time Event Time parameter (index 78).
   // ************************************************************************************************************
   102: XIC(QS18E.Initial_Global_Read)XIO(Command_Being_Processed)XIO(Local_Control.11)EQU(QS18E.Command,48)OTL(Command_Being_Processed)BTD(QS18E.Write_Data.All_Time_Run_Time_Event_Time,24,Port_Data.Data_Transfer[0],0,8)BTD(QS18E.Write_Data.All_Time_Run_Time_Event_Time,16,Port_Data.Data_Transfer[1],0,8)BTD(QS18E.Write_Data.All_Time_Run_Time_Event_Time,8,Port_Data.Data_Transfer[2],0,8)BTD(QS18E.Write_Data.All_Time_Run_Time_Event_Time,0,Port_Data.Data_Transfer[3],0,8)MOV(Port,Port_Data.Data_Transfer[185])MOV(0,Port_Data.Data_Transfer[187])MOV(78,Port_Data.Data_Transfer[188])MOV(4,Port_Data.Data_Transfer[189])MOV(6,Inprocess_Index)OTL(Port_Data.Port_Write.[Port])OTL(Local_Control.11);
   103: NOP();
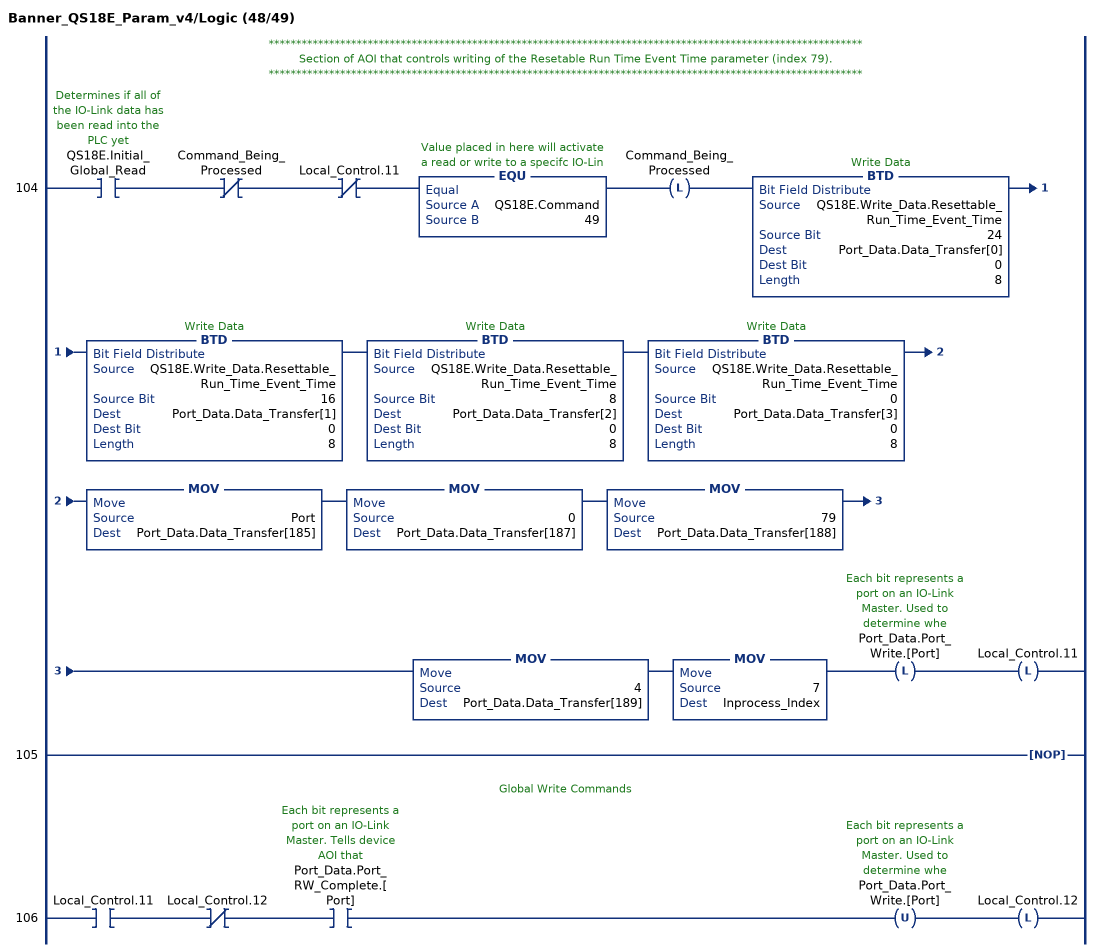
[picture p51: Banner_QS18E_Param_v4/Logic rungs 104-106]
   // ************************************************************************************************************
   // Section of AOI that controls writing of the Resetable Run Time Event Time parameter (index 79).
   // ************************************************************************************************************
   104: XIC(QS18E.Initial_Global_Read)XIO(Command_Being_Processed)XIO(Local_Control.11)EQU(QS18E.Command,49)OTL(Command_Being_Processed)BTD(QS18E.Write_Data.Resettable_Run_Time_Event_Time,24,Port_Data.Data_Transfer[0],0,8)BTD(QS18E.Write_Data.Resettable_Run_Time_Event_Time,16,Port_Data.Data_Transfer[1],0,8)BTD(QS18E.Write_Data.Resettable_Run_Time_Event_Time,8,Port_Data.Data_Transfer[2],0,8)BTD(QS18E.Write_Data.Resettable_Run_Time_Event_Time,0,Port_Data.Data_Transfer[3],0,8)MOV(Port,Port_Data.Data_Transfer[185])MOV(0,Port_Data.Data_Transfer[187])MOV(79,Port_Data.Data_Transfer[188])MOV(4,Port_Data.Data_Transfer[189])MOV(7,Inprocess_Index)OTL(Port_Data.Port_Write.[Port])OTL(Local_Control.11);
   105: NOP();
   // Global Write Commands
   106: XIC(Local_Control.11)XIO(Local_Control.12)XIC(Port_Data.Port_RW_Complete.[Port])OTU(Port_Data.Port_Write.[Port])OTL(Local_Control.12);
